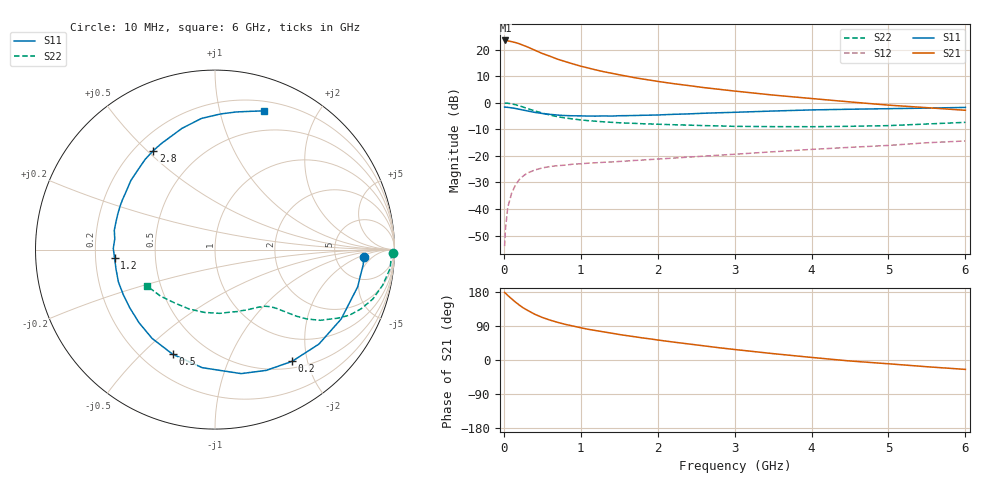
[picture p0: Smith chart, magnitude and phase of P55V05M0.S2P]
! SIEMENS Small Signal Semiconductors
! BFP183
! Si NPN RF Bipolar Junction Transistor in SOT143
! VCE = 5 V  IC = 5 mA
! Common Emitter S-Parameters:  March  1996
# GHz  S  MA  R  50
!  f  S11  S21  S12  S22
! GHz  MAG  ANG  MAG  ANG  MAG  ANG  MAG  ANG
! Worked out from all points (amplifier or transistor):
!   36 points, 10 MHz to 6 GHz, reference 50 ohm
!   highest |S21| = 23.5 dB at 20 MHz (marker M1)
!   |S21| within 3 dB of that: start of sweep to 350.7 MHz
!   unconditionally stable (mu >= 1): 1.607 GHz to 5.69 GHz
!   at 250 MHz: K = 0.20, MSG = 24.6 dB, |S12| = -27.6 dB
!   at 1.4 GHz: K = 0.93, MSG = 16.7 dB, |S12| = -22.3 dB
!   at 6 GHz: K = 0.94, MSG = 5.8 dB, |S12| = -14.4 dB
!   lowest NFmin = 1.15 dB at 450 MHz
!   S11 on the Smith chart (normalised r, x): 10 MHz: 10, -3; 200 MHz: 0.60, -1.75; 500 MHz: 0.32, -0.62; 1.2 GHz: 0.28, -0.04; 2.8 GHz: 0.27, +0.52; 6 GHz: 0.29, +1.37
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0.01  0.8301 -2.7  14.83 178.2  0.002 84.7  0.9929 -1.2
0.02  0.83 -5.8  14.92 176.6  0.004 84.6  0.9827 -2.4
0.05  0.8216 -14.6  14.69 170.6  0.0106 84.7  0.9817 -6.1
0.1  0.8023 -28.8  14.19 161.6  0.0196 74.5  0.955 -12.0
0.15  0.7826 -42.3  13.62 153.0  0.0282 67.7  0.9213 -17.4
0.2  0.7564 -55.4  12.94 145.1  0.0357 62.6  0.8789 -22.0
0.25  0.731 -67.0  12.12 137.9  0.0417 57.1  0.8338 -26.0
0.3  0.7061 -78.1  11.39 132.0  0.0472 52.8  0.7849 -29.1
0.4  0.6617 -96.2  9.817 120.9  0.0541 46.1  0.7063 -33.9
0.5  0.629 -112.0  8.483 112.3  0.0595 40.6  0.6405 -37.1
0.6  0.6064 -125.4  7.528 105.3  0.0631 37.4  0.5876 -39.2
0.7  0.5871 -136.3  6.615 99.3  0.0656 35.4  0.5475 -40.6
0.9  0.5694 -153.8  5.39 89.6  0.07 31.8  0.4957 -42.7
1.1  0.5621 -168.7  4.509 80.9  0.0731 30.5  0.4609 -44.5
1.2  0.5616 -175.1  4.151 77.5  0.0744 30.1  0.4495 -45.5
1.7  0.5768 159.9  2.971 61.4  0.0822 30.3  0.41 -51.3
2.2  0.6066 140.6  2.3 47.4  0.0909 30.9  0.3866 -58.6
2.8  0.6497 122.0  1.794 32.3  0.1033 31.2  0.3674 -70.0
3.5  0.7003 105.2  1.399 16.8  0.1198 30.4  0.3561 -85.8
4.5  0.7565 87.6  1.039 -2.6  0.145 26.6  0.3609 -113.5
5.5  0.7942 75.9  0.81 -17.8  0.177 22.0  0.3991 -139.5
6  0.819 70.7  0.723 -24.8  0.1914 18.1  0.4287 -151.6
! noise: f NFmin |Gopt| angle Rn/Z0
0.45  1.15  0.25  40  0.26
0.9  1.2  0.25  93  0.22
1.8  1.95  0.32  170  0.13
